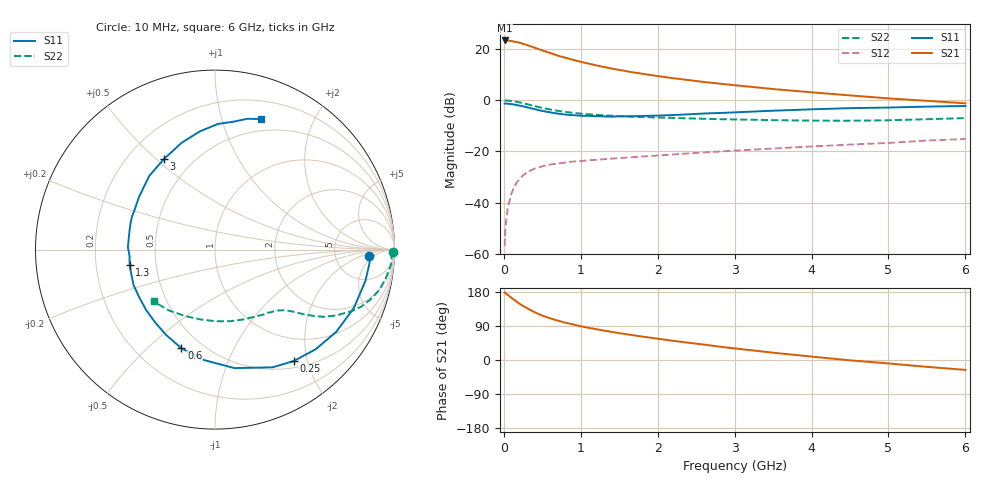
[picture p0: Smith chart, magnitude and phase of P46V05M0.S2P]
! SIEMENS Small Signal Semiconductors
! BFP182
! Si NPN RF Bipolar Junction Transistor in SOT143
! VCE = 6 V  IC = 5 mA
! Common Emitter S-Parameters:  March  1996
# GHz  S  MA  R  50
!  f  S11  S21  S12  S22
! GHz  MAG  ANG  MAG  ANG  MAG  ANG  MAG  ANG
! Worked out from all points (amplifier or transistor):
!   36 points, 10 MHz to 6 GHz, reference 50 ohm
!   highest |S21| = 23.4 dB at 10 MHz (marker M1)
!   |S21| within 3 dB of that: start of sweep to 416.3 MHz
!   unconditionally stable (mu >= 1): 1.646 GHz to 5.588 GHz
!   at 250 MHz: K = 0.21, MSG = 25.7 dB, |S12| = -29.4 dB
!   at 1.4 GHz: K = 0.92, MSG = 17.6 dB, |S12| = -22.9 dB
!   at 6 GHz: K = 0.96, MSG = 7.0 dB, |S12| = -15.2 dB
!   lowest NFmin = 1.20 dB at 450 MHz
!   S11 on the Smith chart (normalised r, x): 10 MHz: 12, -3; 250 MHz: 0.60, -1.77; 600 MHz: 0.39, -0.64; 1.3 GHz: 0.35, -0.08; 3 GHz: 0.35, +0.53; 6 GHz: 0.37, +1.35
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0.01  0.8585 -2.3  14.76 178.3  0.0014 82.0  0.9912 -0.9
0.02  0.8648 -4.7  14.75 177.1  0.0032 85.0  0.9851 -1.9
0.05  0.8563 -11.7  14.7 171.8  0.0078 86.0  0.9847 -4.8
0.1  0.8391 -22.8  14.36 164.0  0.0152 76.7  0.9652 -9.4
0.15  0.8165 -34.1  13.85 156.4  0.0224 71.7  0.9422 -13.9
0.2  0.7889 -44.8  13.42 149.1  0.0283 67.2  0.9105 -17.7
0.25  0.7602 -54.8  12.69 142.5  0.0339 62.2  0.8746 -21.3
0.3  0.7297 -64.0  12.02 137.0  0.0388 58.4  0.8372 -24.1
0.4  0.669 -80.7  10.67 126.1  0.0459 51.7  0.7691 -28.5
0.5  0.6177 -96.1  9.413 117.2  0.051 46.2  0.7104 -31.8
0.6  0.5808 -108.8  8.435 110.1  0.0552 42.9  0.6603 -34.0
0.7  0.5481 -119.8  7.464 104.0  0.0577 40.4  0.6216 -35.7
0.8  0.5244 -129.8  6.79 98.6  0.0604 38.0  0.5912 -36.9
1.1  0.495 -156.3  5.219 84.9  0.067 34.9  0.5314 -39.9
1.3  0.4833 -169.8  4.473 77.7  0.0703 34.0  0.5068 -41.8
1.7  0.4876 167.5  3.472 64.8  0.0776 33.0  0.4754 -46.3
2.2  0.5142 145.7  2.697 50.6  0.087 32.4  0.4519 -53.2
3  0.5793 119.4  1.967 30.6  0.1035 30.7  0.4212 -67.2
3.5  0.6242 107.2  1.655 19.3  0.1136 28.5  0.4081 -77.6
4.5  0.7006 88.6  1.244 -0.9  0.1359 23.8  0.3975 -101.8
5.5  0.7504 76.2  0.973 -18.1  0.163 18.8  0.4258 -127.3
6  0.7719 70.5  0.871 -26.1  0.1745 14.8  0.4474 -139.8
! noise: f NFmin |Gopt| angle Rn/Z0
0.45  1.2  0.27  37  0.3
0.9  1.3  0.25  75  0.23
1.8  1.9  0.21  145  0.2
